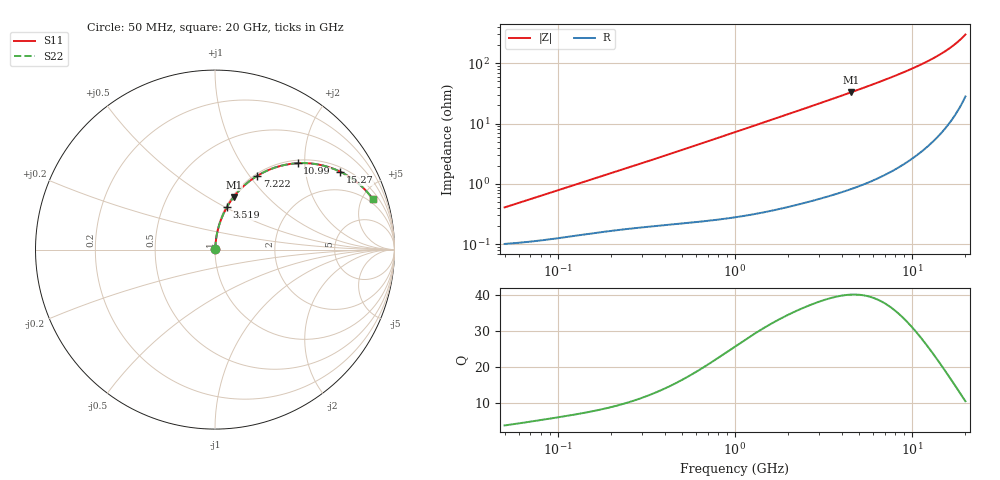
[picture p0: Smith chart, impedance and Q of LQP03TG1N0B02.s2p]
!Murata Part Number: LQP03TG1N0B02
!These Parameters are Measured in Series Mode Connection
!  o--[Z]--o
!Port1  Port2
!  o-------o
!Freq. Start=50[MHz] Stop=20[GHz], 401[Steps]
# Hz S RI R 50
!Freq.(Hz) S11(Real) S11(Imag) S21(Real) S21(Imag) S12(Real) S12(Imag) S22(Real) S22(Imag)
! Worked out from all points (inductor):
!   401 points, 50 MHz to 20 GHz, reference 50 ohm
!   read as one part in series: L = 1.25 nH near 51.52 MHz
!   highest Q = 40.1 at 4.54 GHz (marker M1), where L = 1.16 nH
!   S11 on the Smith chart (normalised r, x): 50 MHz: 1.00, +0.01; 3.519 GHz: 1.01, +0.51; 7.222 GHz: 1.03, +1.09; 10.99 GHz: 1.06, +1.84; 15.27 GHz: 1.16, +3.11; 20 GHz: 1.56, +5.95
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5e7  0.00103 0.00394  0.999 -0.00394  0.999 -0.00394  0.00103 0.00394
1.364002e8  0.00154 0.0104  0.9985 -0.0104  0.9985 -0.0104  0.00154 0.0104
3.721004e8  0.00276 0.0271  0.9972 -0.0271  0.9972 -0.0271  0.00276 0.0271
6.380365e8  0.00447 0.0458  0.9955 -0.0458  0.9955 -0.0458  0.00447 0.0458
1e9  0.00788 0.0711  0.9921 -0.0711  0.9921 -0.0711  0.00788 0.0711
1.714689e9  0.0184 0.1202  0.9816 -0.1202  0.9816 -0.1202  0.0184 0.1202
2.728004e9  0.0415 0.1866  0.9585 -0.1866  0.9585 -0.1866  0.0415 0.1866
3.519108e9  0.0657 0.2353  0.9343 -0.2353  0.9343 -0.2353  0.0657 0.2353
4.539627e9  0.1041 0.2932  0.8959 -0.2932  0.8959 -0.2932  0.1041 0.2932
5.769027e9  0.1599 0.3541  0.8401 -0.3541  0.8401 -0.3541  0.1599 0.3541
7.222371e9  0.2364 0.4117  0.7636 -0.4117  0.7636 -0.4117  0.2364 0.4117
7.442007e9  0.2487 0.4189  0.7513 -0.4189  0.7513 -0.4189  0.2487 0.4189
9.041845e9  0.3425 0.4598  0.6575 -0.4598  0.6575 -0.4598  0.3425 0.4598
1.098561e10  0.4604 0.4813  0.5396 -0.4813  0.5396 -0.4813  0.4604 0.4813
1.295331e10  0.5759 0.474  0.4241 -0.474  0.4241 -0.474  0.5759 0.474
1.417136e10  0.6425 0.4566  0.3575 -0.4566  0.3575 -0.4566  0.6425 0.4566
1.527346e10  0.6983 0.4337  0.3017 -0.4337  0.3017 -0.4337  0.6983 0.4337
1.646126e10  0.7529 0.4027  0.2471 -0.4027  0.2471 -0.4027  0.7529 0.4027
1.747767e10  0.7946 0.3719  0.2054 -0.3719  0.2054 -0.3719  0.7946 0.3719
1.855685e10  0.8338 0.3359  0.1662 -0.3359  0.1662 -0.3359  0.8338 0.3359
1.940974e10  0.861 0.3054  0.139 -0.3054  0.139 -0.3054  0.861 0.3054
2e10  0.8779 0.2836  0.1221 -0.2836  0.1221 -0.2836  0.8779 0.2836
